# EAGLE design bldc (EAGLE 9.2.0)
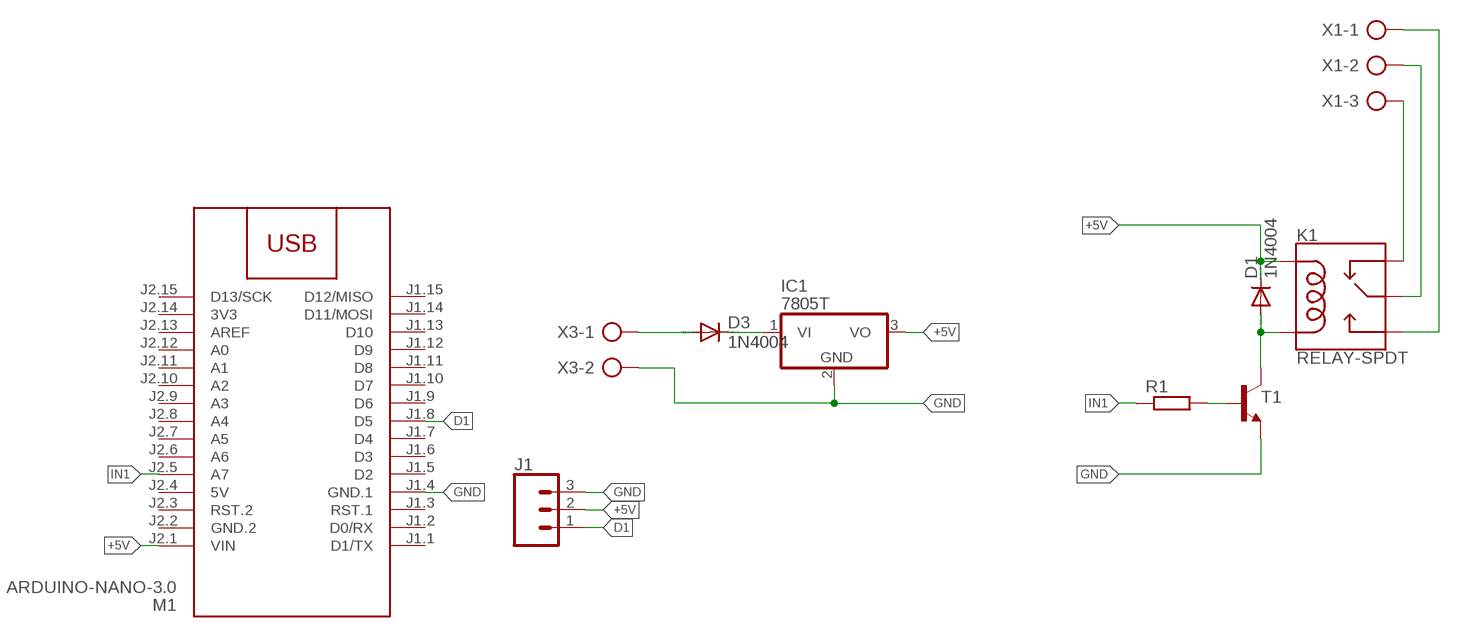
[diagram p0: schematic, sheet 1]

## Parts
D1  1N4004  [DO41-10]
D3  1N4004  [DO41-10]
IC1  7805T  [TO220H]
J1  CONN_03LONGPADS  [1X03_LONGPADS]
K1  RELAY-SPDT  [RELAY_G5LE]
M1  ARDUINO-NANO-3.0  [ARDUINO-NANO-3.0]
R1  R-EU_0207/10  [0207/10]
T1  BC547-NPN-TO92-CBE  [TO92-CBE]
X1  AK300/3  [AK300/3]
X3  AK300/2  [AK300/2]

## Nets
+5V: D1.C IC1.3(VO) J1.2 K1.2(COIL1) M1.J2.1(VIN)
D1: J1.1 M1.J1.8(D5)
GND: IC1.2(GND) J1.3 M1.J1.4(GND.1) T1.E X3.2
IN1: M1.J2.5(A7) R1.1
N$1: K1.4(NC) X1.3
N$2: D1.A K1.5(COIL2) T1.C
N$3: R1.2 T1.B
N$4: K1.1(MAIN) X1.2
N$5: K1.3(NO) X1.1
N$10: D3.C IC1.1(VI)
N$11: D3.A X3.1
Unconnected: M1.J1.1(D1/TX) M1.J1.2(D0/RX) M1.J1.3(RST.1) M1.J1.5(D2) M1.J1.6(D3) M1.J1.7(D4) M1.J1.9(D6) M1.J1.10(D7) M1.J1.11(D8) M1.J1.12(D9) M1.J1.13(D10) M1.J1.14(D11/MOSI) M1.J1.15(D12/MISO) M1.J2.3(RST.2) M1.J2.6(A6) M1.J2.7(A5) M1.J2.8(A4) M1.J2.9(A3) M1.J2.10(A2) M1.J2.11(A1) M1.J2.12(A0) M1.J2.13(AREF) M1.J2.15(D13/SCK)

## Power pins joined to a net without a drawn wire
3V3: M1.J2.14(3V3)
5V: M1.J2.4(5V)
GND.2: M1.J2.2(GND.2)

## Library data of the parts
D1 D3 = diode:1N4004: DIODE
IC1 = linear:78*: Positive VOLTAGE REGULATOR Source: http://cache.national.com/ds/LM/LM78L05.pdf http://www.fairchildsemi.com/ds/LM/LM7805.pdf
J1 = SparkFun-Connectors:CONN_03: Multi connection point. Often used as Generic Header-pin footprint for 0.1 inch spaced/style header connections On any of the 0.1 inch spaced packages, you can populate with these: Break Away Headers - Straight (PRT-00116) Break Away Male Headers - Right Angle (PRT-00553) Female Headers (PRT-00115)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
K1 = SparkFun-Electromechanical:RELAY-SPDT: SPDT Electromechanical Relay Single-pole, double-throw sealed relays. When current is applied to the coil, it throws a simple changeover switch, terminating the connection from the NC contact to ground and closing the NO contact. Use them to switch high voltage/high current devices. SparkFun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; PROD_ID: COMP-14214
M1 = diy-modules:ARDUINO-NANO-3.0: Arduino Nano 3.0 and compatible devices More details available here: https://www.arduino.cc/en/Main/ArduinoBoardNano Click here to find device on ebay.com
R1 = rcl:R-EU_: RESISTOR, European symbol; SPICEPREFIX: R
T1 = transistor:*-NPN-: NPN Transistror BF959 corrected 2008.03.06
X1 = con-ptr500:AK300/3: CONNECTOR; OC_FARNELL: unknown; OC_NEWARK: unknown
X3 = con-ptr500:AK300/2: CONNECTOR; OC_FARNELL: unknown; OC_NEWARK: unknown

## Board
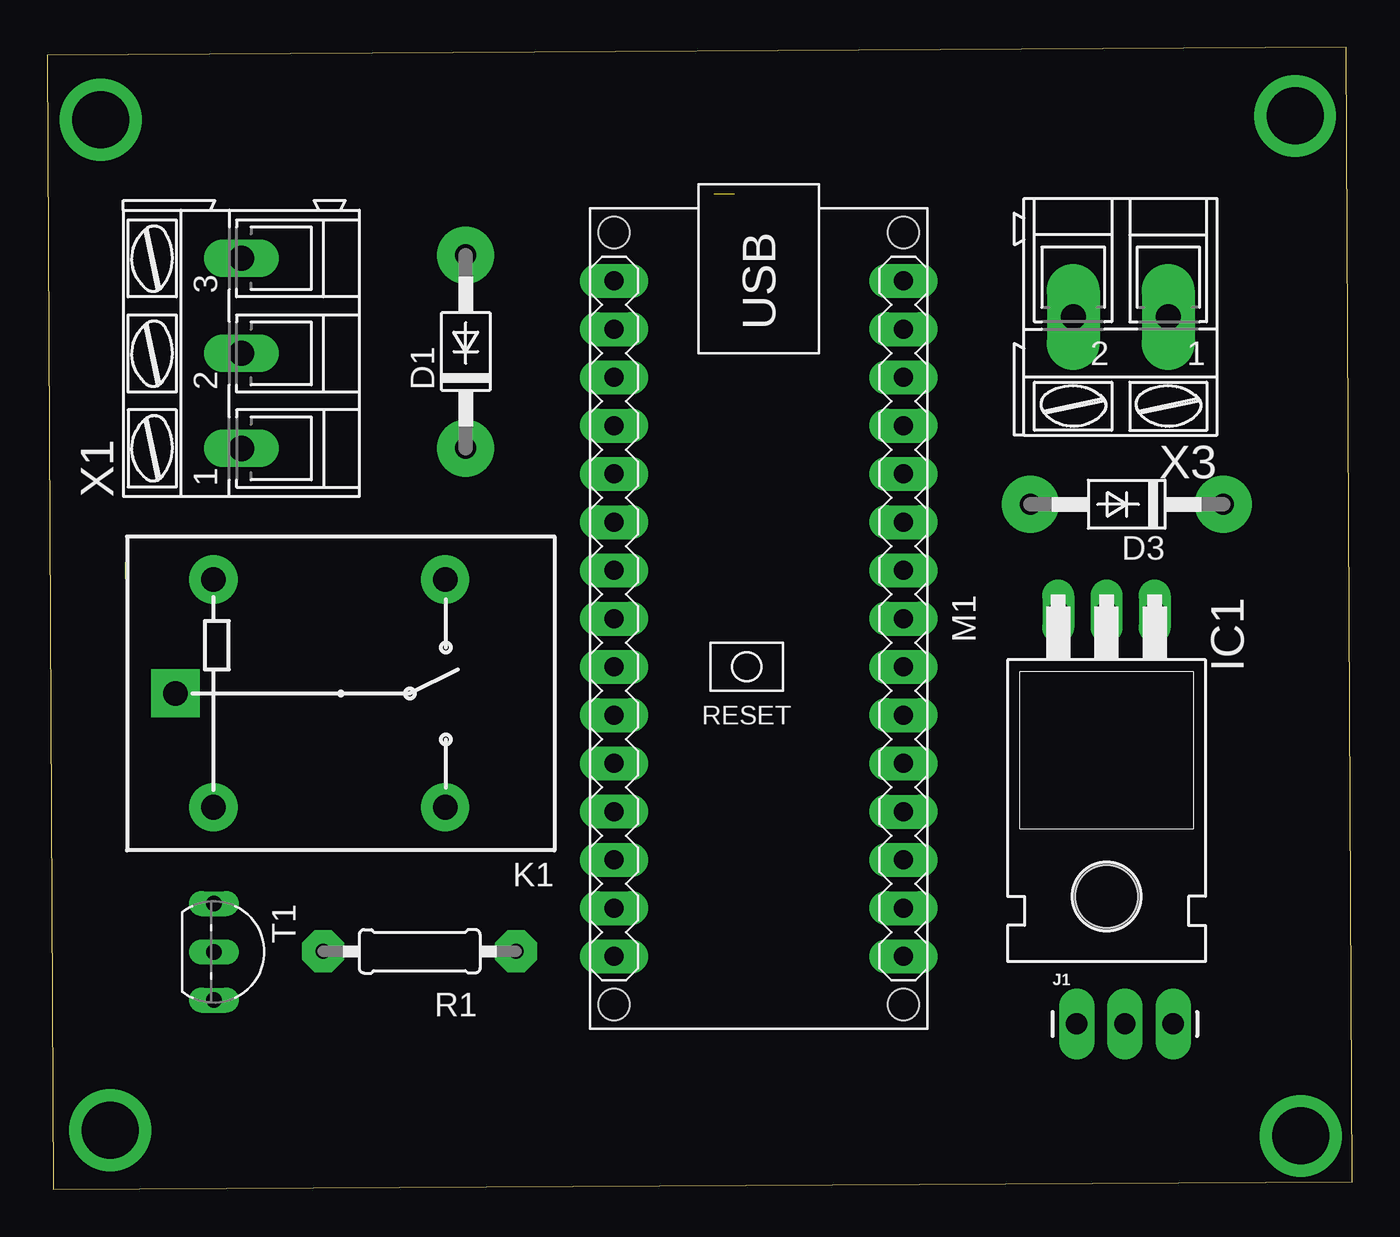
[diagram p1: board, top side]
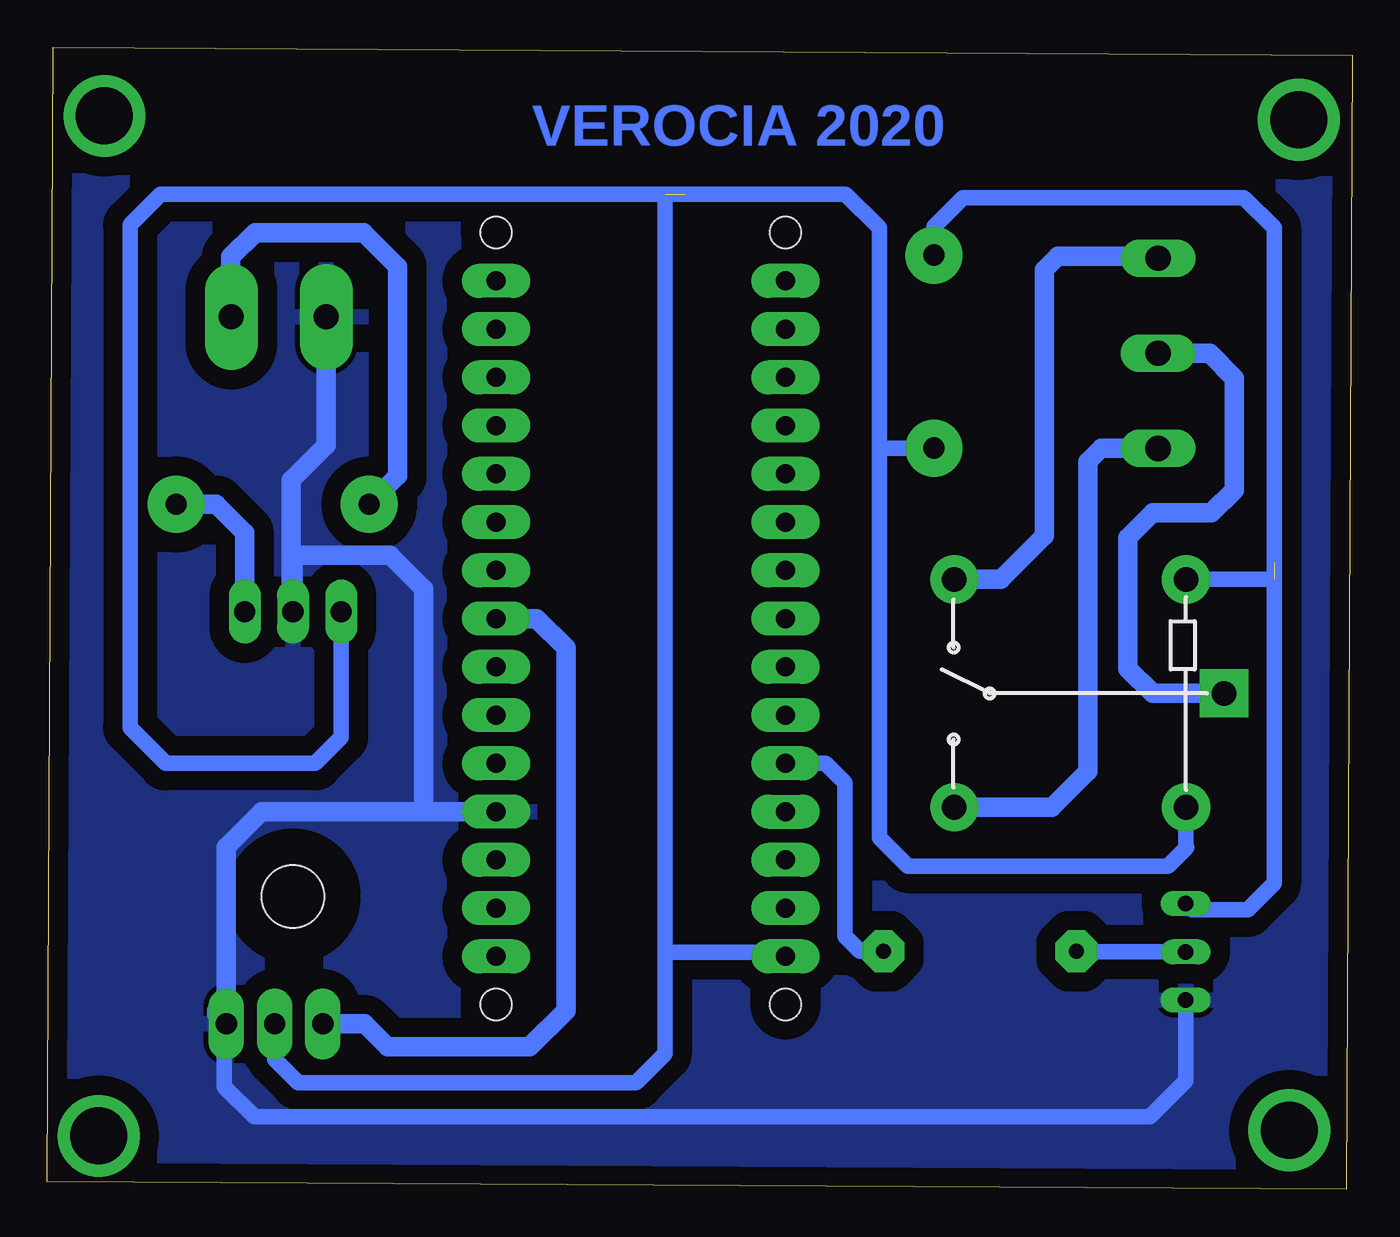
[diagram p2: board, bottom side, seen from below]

Size 68.7 x 60.1 mm. Coordinates in mm from the lower left corner, seen from the top.
Outline: 0.3,0 68.7,0.4 68.4,60.1 0,59.7 0.3,0
Copper layers (1*16): Top 0.035mm / dielectric 1.5mm / Bottom 0.035mm
Design rules "default": minimum track width 6mil, minimum drill 0.35mm, track to track 6mil, track to pad 6mil, pad to pad 6mil, via to via 6mil, smd to smd 6mil, copper to edge 40mil, drill to drill 6mil, minimum pad ring 10mil, minimum via ring 8mil, stop-mask expansion 4mil, vias tented up to drill 0mil, thermal gap 10mil

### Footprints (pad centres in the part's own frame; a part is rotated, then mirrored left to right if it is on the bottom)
DO41-10 = drill 1.118 pad 3: A 5.08,0; C -5.08,0
TO220H = drill 1.118 long: 1 -2.54,-10.16; 2 0,-10.16; 3 2.54,-10.16 | hole 3.302: 0,4.826
1X03_LONGPADS = drill 1.118 pad 1.88 long: 1 0,0; 2 2.54,0; 3 5.08,0
RELAY_G5LE = drill 1.3 pad 2.54 square: 1 8.52,-0.005 | drill 1.3 pad 2.54: 2 6.52,5.995; 3 -5.68,5.995; 4 -5.68,-6.005; 5 6.52,-6.005
ARDUINO-NANO-3.0 = drill 1 pad 1.8 long: J1.1 17.78,7.62; J1.2 15.24,7.62; J1.3 12.7,7.62; J1.4 10.16,7.62; J1.5 7.62,7.62; J1.6 5.08,7.62; J1.7 2.54,7.62; J1.8 0,7.62; J1.9 -2.54,7.62; J1.10 -5.08,7.62; J1.11 -7.62,7.62; J1.12 -10.16,7.62; J1.13 -12.7,7.62; J1.14 -15.24,7.62; J1.15 -17.78,7.62; J2.1 17.78,-7.62; J2.2 15.24,-7.62; J2.3 12.7,-7.62; J2.4 10.16,-7.62; J2.5 7.62,-7.62; J2.6 5.08,-7.62; J2.7 2.54,-7.62; J2.8 0,-7.62; J2.9 -2.54,-7.62; J2.10 -5.08,-7.62; J2.11 -7.62,-7.62; J2.12 -10.16,-7.62; J2.13 -12.7,-7.62; J2.14 -15.24,-7.62; J2.15 -17.78,-7.62 | hole 1.651: -20.32,7.62; -20.32,-7.62; 20.32,-7.62; 20.32,7.62
0207/10 = drill 0.8 pad 2.2 octagon: 1 -5.08,0; 2 5.08,0
TO92-CBE = drill 0.813 long: B 0,0; C -2.54,0; E 2.54,0
AK300/3 = drill 1.321 long: 1 -5.004,0; 2 0,0; 3 5.004,0
AK300/2 = drill 1.321 pad 2.8 long: 1 -2.515,0; 2 2.489,0

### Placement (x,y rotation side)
D1  22.03,44.09 90 top
D3  56.83,36.05 180 top
IC1  55.77,20.24 180 top
J1  54.2,8.7 0 top
K1  15.27,26.09 180 top
M1  37.45,30.04 270 top
R1  19.6,12.52 180 top
T1  8.76,12.49 270 top
X1  10.21,43.99 90 top
X3  56.5,45.91 180 top

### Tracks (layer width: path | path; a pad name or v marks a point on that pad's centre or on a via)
+5V  (1 unrouted)
  Bottom 0.813: M1.J2.1 30.04,12.46 36.11,12.46 36.18,12.53 | 35.1,52.37 62.74,52.37 64.36,50.76 64.36,24.29 62.48,22.42 54.6,22.42 53.23,23.79 IC1.3 | 36.18,12.53 36.18,52.37 26.67,52.37 24.9,50.6 24.9,39.02 | 24.9,39.02 D1.C | J1.2 56.74,6.84 55.5,5.6 37.7,5.6 36.18,7.12 36.18,12.53 | 24.9,39.02 24.9,18.5 23.4,17 9.7,17 8.7,18 8.75,18.05 K1.2
D1
  Bottom 1.016: J1.1 52,8.7 50.8,7.5 43.3,7.5 41.4,9.4 41.4,28.5 42.94,30.04 M1.J1.8
GND
  Bottom 0.813: T1.E 8.76,5.7 10.66,3.8 57.8,3.8 59.4,5.4 59.4,8.58 J1.3
  Bottom 1.016: X3.2 54.02,39.17 55.87,37.31 55.87,30.68 55.77,30.68 | 55.77,30.68 55.77,33.38 50.65,33.38 48.88,31.61 48.88,19.88 | 55.77,30.68 IC1.2 | 48.88,19.88 M1.J1.4 | 59.8,9.4 59.8,9.22 J1.3 59.28,11.38 59.3,11.4 59.3,18 57.42,19.88 48.88,19.88
  pour Bottom (isolate 1.016): 0,59.7 68.9,59.7 68.9,0.1 0,0.1
IN1
  Bottom 0.813: R1.1 25.92,12.52 26.7,13.3 26.7,21.39 27.73,22.42 M1.J2.5
N$1
  Bottom 1.016: K1.4 18.5,32.1 16.2,34.4 16.2,48.4 15.5,49.1 10.32,49.1 X1.3
N$2  (1 unrouted)
  Bottom 0.813: K1.5 4.1,32.1 4.1,50.6 5.7,52.2 20.5,52.2 22.03,50.67 D1.A | 4.1,33 4.1,16.1 5.5,14.7 8.43,14.7 T1.C
N$3
  Bottom 0.813: T1.B 14.49,12.49 R1.2
N$4
  Bottom 1.016: K1.1 10.5,26.1 11.8,27.4 11.8,34.3 10.5,35.6 7.4,35.6 6.2,36.8 6.2,42.7 7.5,43.99 X1.2
N$5
  Bottom 1.016: X1.1 13.21,38.99 13.9,38.3 13.9,22 15.8,20.1 K1.3
N$6  (via drill 3 pad 4.3)
  other vias: 65.7,56.5
N$7  (via drill 3 pad 4.3)
  other vias: 3.3,3.1
N$10
  Bottom 1.016: D3.C 59.81,36.05 58.31,34.55 IC1.1
N$11
  Bottom 1.016: D3.A 50.25,37.55 50.25,48.55 52.06,50.36 57.77,50.36 59.04,49.09 59.04,45.94 X3.1
N$14  (via drill 3 pad 4.3)
  other vias: 66,2.8
Q  (via drill 3 pad 4.3)
  other vias: 2.8,56.3

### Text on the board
Bottom: VEROCIA 2020

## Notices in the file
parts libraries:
diy-modules: Released under the Creative Commons Attribution 4.0 International License: http://creativecommons.org/licenses/by/4.0
SparkFun-Electromechanical: Licensing: Creative Commons ShareAlike 4.0 International - https://creativecommons.org/licenses/by-sa/4.0
